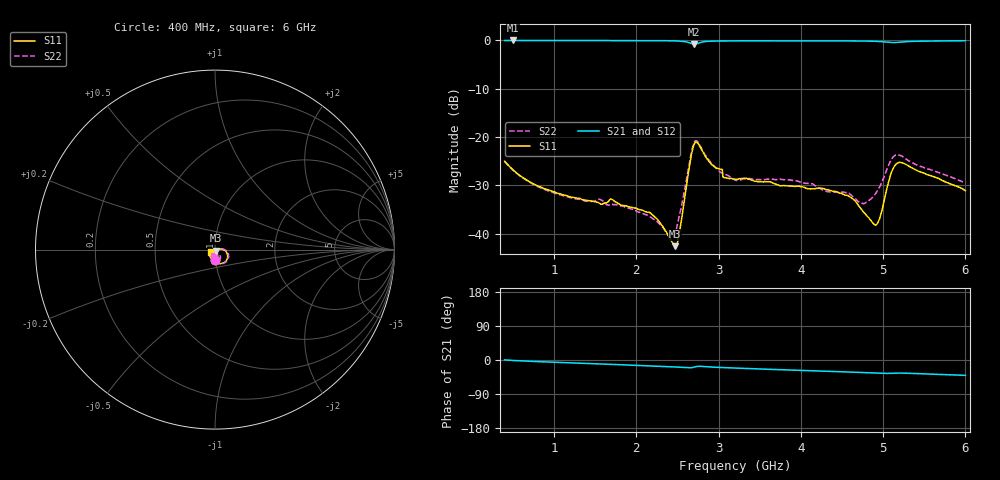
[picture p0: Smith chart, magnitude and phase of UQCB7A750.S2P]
!  Part Number  UQCB7A750	Mounting Orientation: Vertical
!  Description: RF capacitors
!  Application: Coupling, Bypass, Tuning, DC Block
!  Filters, Matching
# GHZ S DB R 50
! Freq  |S11|  S11 Ph  |S21|  S21 Ph  |S12|  S12 Ph  |S22|  S22 Ph
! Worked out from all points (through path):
!   801 points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, 400 MHz to 6 GHz, reference 50 ohm
!   highest |S21| = -0.03 dB at 505 MHz (marker M1); lowest = -0.8 dB at 2.703 GHz (marker M2)
!   group delay of S21, straight-line fit = 19.3 ps
!   lowest |S11| = -42.6 dB at 2.472 GHz (marker M3), VSWR 1.01, Z = 50.5 - j0.58 ohm
!   |S11| at or under -10 dB: start of sweep to end of sweep
!   |S22| runs from -40.7 to -20.8 dB; largest |S21 - S12| = 0.0025
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0.4  -25.01 -88.5  -0.03 0.2  -0.02 0.2  -25.02 -88.0
0.505  -26.87 -89.4  -0.03 -1.2  -0.02 -1.2  -26.88 -88.6
0.834  -30.32 -91.9  -0.03 -4.5  -0.02 -4.6  -30.52 -90.0
1.338  -32.90 -98.0  -0.04 -8.7  -0.03 -8.8  -33.01 -90.5
1.709  -32.94 -101.0  -0.05 -11.6  -0.04 -11.7  -33.93 -90.3
2.269  -37.28 -101.9  -0.07 -16.2  -0.06 -16.2  -37.76 -81.1
2.402  -40.76 -83.7  -0.10 -17.5  -0.09 -17.5  -40.66 -55.8
2.472  -42.58 -50.7  -0.12 -18.3  -0.11 -18.3  -40.01 -21.9
2.521  -40.06 -13.0  -0.16 -18.9  -0.15 -19.0  -36.41 -2.5
2.654  -25.23 -5.0  -0.55 -20.6  -0.54 -20.7  -24.52 -3.3
2.703  -21.50 -34.1  -0.82 -18.8  -0.81 -18.9  -21.14 -31.2
3.081  -28.43 -105.2  -0.14 -20.2  -0.13 -20.3  -27.80 -93.1
3.2  -28.74 -109.0  -0.12 -21.1  -0.11 -21.2  -28.92 -96.0
4.138  -30.69 -132.4  -0.13 -28.3  -0.12 -28.3  -29.67 -113.1
4.586  -32.27 -140.2  -0.13 -31.8  -0.12 -31.9  -31.67 -102.8
4.754  -35.36 -137.2  -0.16 -33.0  -0.15 -33.1  -33.77 -86.2
4.908  -38.23 -101.1  -0.20 -34.5  -0.20 -34.6  -31.71 -59.6
4.964  -36.50 -76.3  -0.26 -35.0  -0.26 -35.1  -30.13 -52.7
5.069  -29.09 -66.3  -0.43 -35.3  -0.42 -35.4  -25.72 -54.0
5.139  -25.98 -84.4  -0.47 -34.7  -0.46 -34.8  -23.88 -68.8
5.216  -25.27 -105.2  -0.36 -34.5  -0.35 -34.5  -23.86 -84.8
6  -31.10 -148.3  -0.09 -40.5  -0.09 -40.6  -29.46 -99.1
